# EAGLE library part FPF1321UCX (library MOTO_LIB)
SPDT Power switch. Reverse blocking.
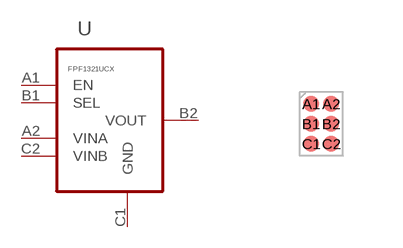
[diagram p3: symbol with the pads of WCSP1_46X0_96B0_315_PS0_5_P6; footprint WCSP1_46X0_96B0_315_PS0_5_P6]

Designator prefix U

## FPF1321UCX (MPN: FPF1321UCX; SUPPLIER: FAIRCHILD)  [WCSP1_46X0_96B0_315_PS0_5_P6]
A1  EN  in
A2  VINA  pwr
B1  SEL  in
B2  VOUT  in
C1  GND  in
C2  VINB  pwr

## Footprint WCSP1_46X0_96B0_315_PS0_5_P6 (pad centres in mm)
smd 0.4 x 0.4: A1 -0.25,0.5; A2 0.25,0.5; B1 -0.25,0; B2 0.25,0; C1 -0.25,-0.5; C2 0.25,-0.5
